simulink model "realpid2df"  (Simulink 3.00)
settings: Solver=ode45  SolverMode=SingleTasking  StartTime=0.0  StopTime=10  FixedStep=st_size  MaxStep=st_size  RelTol=1e-5  AbsTol=1e-6
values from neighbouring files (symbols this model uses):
  d_through_p = get(MAIN_MENU(19),'Value')    [cback.m]    (also in imcmenu.m = 0)
  Disturb = Setpoint    [mimo_MSF1DF_sim.m]    (also in mimo_MSF2DF_sim.m)
  K = 1/kpd    [imc2pseucon.m]    (also in imc2pseudo.m)
  Satlb = temp1    [cback.m]    (also in imcmenu.m = str2num(satlbs))
  Satub = temp1    [cback.m]    (also in imcmenu.m = str2num(satubs))
  Setpoint = zeros(1,n)    [mimo_MSF1DF_sim.m]    (also in mimo_MSF2DF_sim.m)
undefined symbols (not defined in the file or in its folder): denPd, denPs, numPd, numPs, Pre_fil_den, Pre_fil_num, TauD, TauI
libraries: MIMO_lib x1

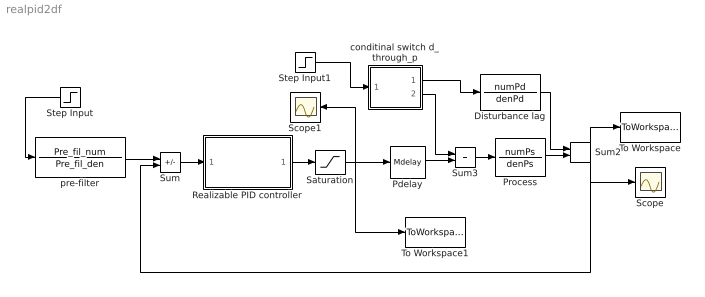
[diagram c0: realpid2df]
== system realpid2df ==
  Disturbance lag : TransferFcn  Numerator=numPd  Denominator=denPd
  Pdelay : MIMO_lib/Mdelay  Mdelay=Pdelay
  Process : TransferFcn  Numerator=numPs  Denominator=denPs
  Realizable PID controller : Subsystem
  Saturation : Saturate  UpperLimit=Satub  LowerLimit=Satlb
  Scope : Scope
  Scope1 : Scope
  Step Input : Step  Orientation=left  Time=0  Before=0  After=Setpoint  SampleTime=0
  Step Input1 : Step  Time=0  Before=0  After=Disturb  SampleTime=0
  Sum : Sum  Inputs=+-  SaturateOnIntegerOverflow=on
  Sum2 : Sum  Inputs=++  SaturateOnIntegerOverflow=on
  Sum3 : Sum  Inputs=++  SaturateOnIntegerOverflow=on
  To Workspace : ToWorkspace  VariableName=simout  SampleTime=-1  SaveFormat=Matrix
  To Workspace1 : ToWorkspace  VariableName=effort  SampleTime=-1  SaveFormat=Matrix
  conditinal switch d_through_p : Subsystem  Description=pass input signal through out1 if condition is true.
  pre-filter : TransferFcn  Numerator=Pre_fil_num  Denominator=Pre_fil_den
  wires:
  pre-filter/1 -> Sum/1
  Sum/1 -> Realizable PID controller/1(In1)
  Step Input/1 -> pre-filter/1
  Realizable PID controller/1(Out1) -> Saturation/1
  Pdelay/1 -> Sum3/2
  Sum3/1 -> Process/1
  Process/1 -> Sum2/2
  Disturbance lag/1 -> Sum2/1
  conditinal switch d_through_p/2(Out1) -> Sum3/1
  conditinal switch d_through_p/1(Out2) -> Disturbance lag/1
  Step Input1/1 -> conditinal switch d_through_p/1(In)
  Saturation/1 -> Pdelay/1, Scope1/1, To Workspace1/1
  Sum2/1 -> Sum/2, To Workspace/1, Scope/1

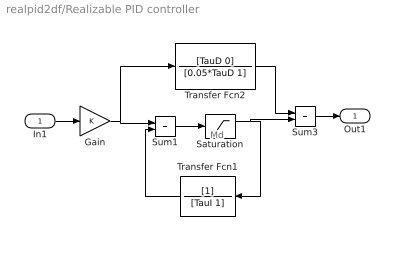
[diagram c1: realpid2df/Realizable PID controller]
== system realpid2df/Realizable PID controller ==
  note: Md
  In1 : Inport  Port=1  PortWidth=-1  SampleTime=-1  DataType=auto
  Gain : Gain  Gain=K  SaturateOnIntegerOverflow=on
  Saturation : Saturate  UpperLimit=Satub  LowerLimit=Satlb
  Sum1 : Sum  Inputs=++  SaturateOnIntegerOverflow=on
  Sum3 : Sum  Inputs=++  SaturateOnIntegerOverflow=on
  Transfer Fcn1 : TransferFcn  Orientation=left  Numerator=[1]  Denominator=[TauI 1]
  Transfer Fcn2 : TransferFcn  Numerator=[TauD 0]  Denominator=[0.05*TauD 1]
  Out1 : Outport  Port=1  InitialOutput=0
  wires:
  Sum1/1 -> Saturation/1
  Transfer Fcn1/1 -> Sum1/2
  Gain/1 -> Sum1/1, Transfer Fcn2/1
  Saturation/1 -> Transfer Fcn1/1, Sum3/2
  Transfer Fcn2/1 -> Sum3/1
  Sum3/1 -> Out1/1
  In1/1 -> Gain/1

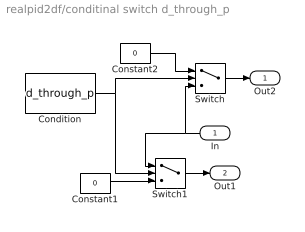
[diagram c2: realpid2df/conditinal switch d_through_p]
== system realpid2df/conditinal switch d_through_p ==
  In : Inport  Orientation=left  Port=1  PortWidth=-1  SampleTime=-1  DataType=auto
  Condition : Constant  Value=d_through_p
  Constant1 : Constant  Value=0
  Constant2 : Constant  Value=0
  Switch : Switch  Threshold=1
  Switch1 : Switch  Threshold=1
  Out2 : Outport  Port=1  InitialOutput=0
  Out1 : Outport  Port=2  InitialOutput=0
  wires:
  In/1 -> Switch/3, Switch1/1
  Condition/1 -> Switch1/2, Switch/2
  Constant1/1 -> Switch1/3
  Constant2/1 -> Switch/1
  Switch/1 -> Out2/1
  Switch1/1 -> Out1/1
